FUNCTION "Var_assign_FC" : Bool
VERSION : 0.1
   VAR_INPUT
      inFC : Bool;
   END_VAR

   VAR_OUTPUT
      outFC : Bool;
   END_VAR

   VAR_IN_OUT
      inoutFC : Bool;
   END_VAR

   VAR_TEMP
      tempFC : Bool;
   END_VAR

   VAR CONSTANT
      constFC : Bool;
   END_VAR


BEGIN
NETWORK
TITLE =
END_FUNCTION

FUNCTION_BLOCK "Var_assign_FB"
VERSION : 0.1
   VAR_INPUT
      "! #$%&'()*+,-./0123456789:;<=>?@ABCDEFGHIJKLMNOPQRSTUVWXYZ[\]^_`abcdefghijklmnopqrstuvwxyz{|}~" : Bool := true;
   END_VAR

   VAR_OUTPUT
      out : Int := 6;
   END_VAR

   VAR_IN_OUT
      inout : Real := 4.5;
   END_VAR

   VAR
      static : DInt := 134142;
   END_VAR

   VAR_TEMP
      temp : Bool;
   END_VAR

   VAR CONSTANT
      "constant" : Bool;
   END_VAR


BEGIN
NETWORK
TITLE =
END_FUNCTION_BLOCK

